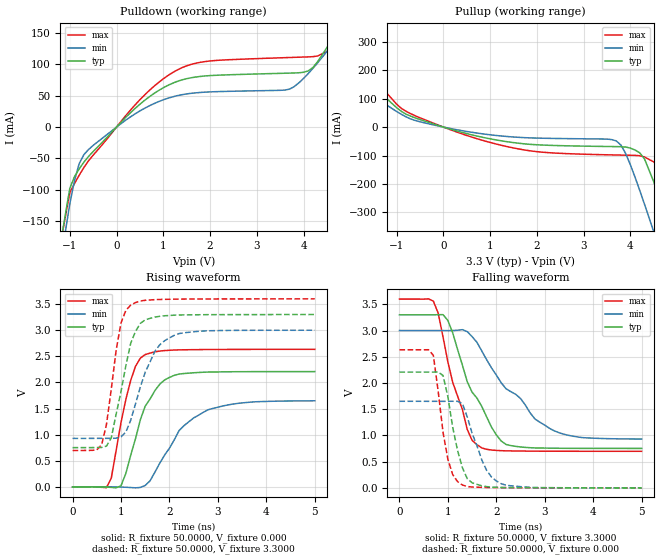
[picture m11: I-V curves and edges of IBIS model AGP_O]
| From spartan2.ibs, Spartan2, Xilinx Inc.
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|   Model AGP_O
[Model]   AGP_O
Model_type   Output
Polarity   Non-Inverting
| Vmeas depends on rising or falling edge, select one of the following:
| For rising edge:
|Vmeas =   0.940V
| For falling edge:
|Vmeas =   2.00V
Cref =  10.0000pF
Rref =  50.0000
| Vref depends on rising or falling edge, select one of the following:
| For rising edge:
|Vref =   0.00V
| For falling edge:
|Vref =   3.30V
C_comp   6.5000pF   5.0000pF   8.0000pF
[Temperature Range]   27.0000   100.0000   0.000
[Voltage Range]   3.3000V   3.0000V   3.6000V
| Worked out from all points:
|   slope of the pulldown table from 0 to 0.495 V, typ, clamps not added: 13.7 ohm
|   slope of the pullup table from 0 to 0.495 V, typ, clamps not added: 21.7 ohm
|   rising waveform, R_fixture 50.0000, V_fixture 0.000: 20-80 % time 499ps typ, 771ps min, 358ps max; typ from 0 V to 2.21 V
|   rising waveform, R_fixture 50.0000, V_fixture 3.3000: 20-80 % time 348ps typ, 473ps min, 265ps max; typ from 0.751 V to 3.3 V
|   falling waveform, R_fixture 50.0000, V_fixture 3.3000: 20-80 % time 695ps typ, 1.06ns min, 488ps max; typ from 3.3 V to 0.752 V
|   falling waveform, R_fixture 50.0000, V_fixture 0.000: 20-80 % time 290ps typ, 392ps min, 245ps max; typ from 2.21 V to 0 V
[Pulldown]
| voltage   I(typ)   I(min)   I(max)
-3.3V     -1.282A    -1.27A     -1.284A
-1.5V     -319.5mA   -354.4mA   -307.2mA
-1V       -97.76mA   -122.6mA   -104.7mA
-800mV    -66.76mA   -58.46mA   -76.88mA
-600mV    -46.93mA   -35.82mA   -53.89mA
500mV     36.44mA    25.74mA    43.59mA
1.4V      75.27mA    51.64mA    94.7mA
3.7V      86.04mA    60.44mA    110.9mA
4.1V      89.49mA    85.22mA    111.9mA
4.5V      126.6mA    120.5mA    120.3mA
4.9V      177.6mA    159.9mA    174.2mA
6.6V      407.8mA    336.3mA    452.6mA
[Pullup]
| voltage   I(typ)   I(min)   I(max)
-3.3V     413.8mA    317.9mA    498.5mA
-2.9V     356.6mA    273mA      429.3mA
-2.5V     297.6mA    226.1mA    358.6mA
-600mV    31.98mA    22.96mA    39.44mA
1.5V      -54.66mA   -34.94mA   -73.46mA
3.7V      -68.75mA   -48.9mA    -98.25mA
3.9V      -70.27mA   -93.43mA   -98.9mA
4.2V      -90.62mA   -222.7mA   -100.8mA
4.5V      -192.3mA   -368.3mA   -122.6mA
4.9V      -393.7mA   -569.2mA   -241mA
5.1V      -499.3mA   -670.9mA   -340.5mA
6.6V      -1.31A     -1.442A    -1.157A
[Ramp]
| variable   typ   min   max
dV/dt_r   1.3242/0.4971n   0.9888/0.7709n   1.5792/0.3468n
dV/dt_f   1.5287/0.6912n   1.2413/1.0958n   1.7416/0.4938n
R_load = 50.0000
[Rising Waveform]
R_fixture = 50.0000
V_fixture = 0.000
| time   V(typ)   V(min)   V(max)
0s        0V         0V         0V
700ps     -3.8mV     862.5uV    -14.13mV
800ps     -9.51mV    982.4uV    170.4mV
1ns       21.17mV    -3.713mV   1.232V
1.3ns     925mV      -18.54mV   2.309V
1.5ns     1.547V     27.03mV    2.533V
2ns       2.096V     739.6mV    2.615V
2.3ns     2.17V      1.172V     2.624V
2.8ns     2.198V     1.478V     2.629V
5ns       2.207V     1.648V     2.632V
[Rising Waveform]
R_fixture = 50.0000
V_fixture = 3.3000
V_fixture_min = 3.0000
V_fixture_max = 3.6000
| time   V(typ)   V(min)   V(max)
0s        751.2mV    928.2mV    696.8mV
600ps     755.2mV    928.8mV    804.3mV
700ps     780.4mV    929mV      1.195V
800ps     939.8mV    928.5mV    1.876V
1ns       1.823V     959.2mV    3.139V
1.2ns     2.746V     1.276V     3.479V
1.4ns     3.13V      1.916V     3.558V
1.7ns     3.25V      2.596V     3.584V
2.1ns     3.287V     2.901V     3.593V
5ns       3.299V     2.999V     3.599V
[Falling Waveform]
R_fixture = 50.0000
V_fixture = 3.3000
V_fixture_min = 3.0000
V_fixture_max = 3.6000
| time   V(typ)   V(min)   V(max)
0s        3.3V       3V         3.6V
700ps     3.299V     3V         3.562V
800ps     3.303V     3V         3.33V
1ns       3.192V     2.999V     2.401V
1.4ns     2.024V     2.98V      1.114V
1.7ns     1.552V     2.61V      761.6mV
2ns       1.011V     2.151V     714.3mV
2.2ns     828.1mV    1.89V      706mV
3.1ns     757.3mV    1.134V     699.1mV
5ns       752.1mV    931.2mV    697.4mV
[Falling Waveform]
R_fixture = 50.0000
V_fixture = 0.000
| time   V(typ)   V(min)   V(max)
0s        2.208V     1.651V     2.633V
700ps     2.208V     1.651V     2.529V
900ps     2.143V     1.65V      1.058V
1ns       1.738V     1.651V     545.8mV
1.1ns     1.153V     1.651V     251.5mV
1.3ns     385.2mV    1.607V     54.49mV
1.5ns     96.57mV    1.042V     16.26mV
1.8ns     23.66mV    334.1mV    8.044mV
2.1ns     8.124mV    79.81mV    4.419mV
5ns       448.4uV    515.5uV    436.4uV
